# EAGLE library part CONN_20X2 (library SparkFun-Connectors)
Multi connection point. Often used as Generic Header-pin footprint for 0.1 inch spaced/style header connections On any of the 0.1 inch spaced packages, you can populate with these: Break Away Headers - Straight (PRT-00116) Break Away Male Headers - Right Angle (PRT-00553) Female Headers (PRT-00115) Break Away Headers - Machine Pin (PRT-00117) Break Away Female Headers - Swiss Machine Pin (PRT-00743)
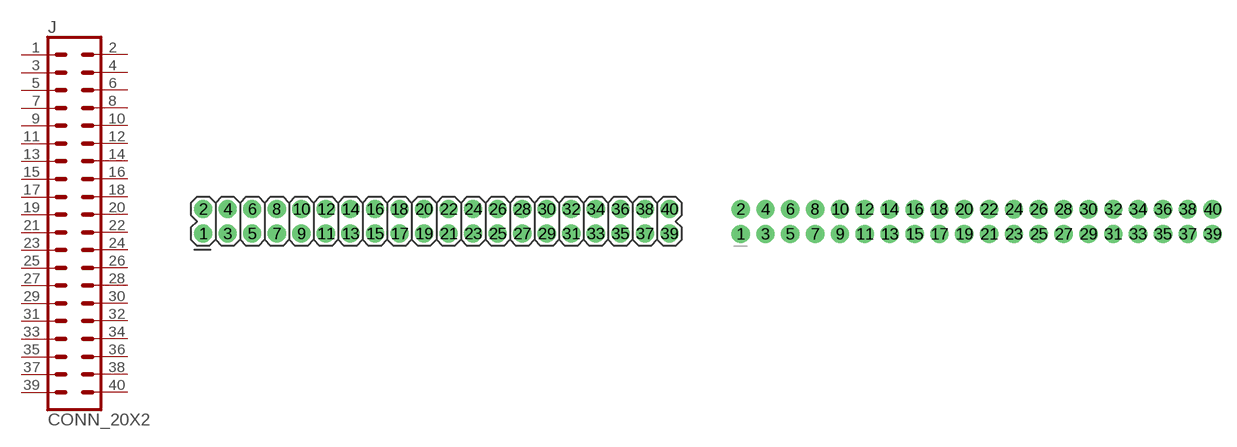
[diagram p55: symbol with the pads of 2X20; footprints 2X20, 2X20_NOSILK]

Designator prefix J

## CONN_20X2  [2X20]
1  1  pas
2  2  pas
3  3  pas
4  4  pas
5  5  pas
6  6  pas
7  7  pas
8  8  pas
9  9  pas
10  10  pas
11  11  pas
12  12  pas
13  13  pas
14  14  pas
15  15  pas
16  16  pas
17  17  pas
18  18  pas
19  19  pas
20  20  pas
21  21  pas
22  22  pas
23  23  pas
24  24  pas
25  25  pas
26  26  pas
27  27  pas
28  28  pas
29  29  pas
30  30  pas
31  31  pas
32  32  pas
33  33  pas
34  34  pas
35  35  pas
36  36  pas
37  37  pas
38  38  pas
39  39  pas
40  40  pas

## CONN_20X2NOSILK  [2X20_NOSILK]
Pads as for 2X20

## CONN_20X2SHROUDED (PROD_ID: CONN-12263; SF_ID: CONN-12263)  [2X20_SHROUDED]
Pads as for 2X20

## CONN_20X2SHROUDED_SMT (PROD_ID: CONN-13143)  [2X20_SHROUDED_SMT]
Pads as for 2X20

## Footprint 2X20 (pad centres in mm)
Plated Through Hole - 2x20 Specifications: Pin count:40 Pin pitch:0.1" Example device(s): CONN_20x2
drill 1.016 pad 1.88: 1 0,0; 2 0,2.54; 3 2.54,0; 4 2.54,2.54; 5 5.08,0; 6 5.08,2.54; 7 7.62,0; 8 7.62,2.54; 9 10.16,0; 10 10.16,2.54; 11 12.7,0; 12 12.7,2.54; 13 15.24,0; 14 15.24,2.54; 15 17.78,0; 16 17.78,2.54; 17 20.32,0; 18 20.32,2.54; 19 22.86,0; 20 22.86,2.54; 21 25.4,0; 22 25.4,2.54; 23 27.94,0; 24 27.94,2.54; 25 30.48,0; 26 30.48,2.54; 27 33.02,0; 28 33.02,2.54; 29 35.56,0; 30 35.56,2.54; 31 38.1,0; 32 38.1,2.54; 33 40.64,0; 34 40.64,2.54; 35 43.18,0; 36 43.18,2.54; 37 45.72,0; 38 45.72,2.54; 39 48.26,0; 40 48.26,2.54

## Footprint 2X20_NOSILK (pad centres in mm)
Plated Through Hole - 2x20 No Silk Outline Specifications: Pin count:40 Pin pitch:0.1" Example device(s): CONN_20x2
drill 1.016 pad 1.88: 1 0,0; 2 0,2.54; 3 2.54,0; 4 2.54,2.54; 5 5.08,0; 6 5.08,2.54; 7 7.62,0; 8 7.62,2.54; 9 10.16,0; 10 10.16,2.54; 11 12.7,0; 12 12.7,2.54; 13 15.24,0; 14 15.24,2.54; 15 17.78,0; 16 17.78,2.54; 17 20.32,0; 18 20.32,2.54; 19 22.86,0; 20 22.86,2.54; 21 25.4,0; 22 25.4,2.54; 23 27.94,0; 24 27.94,2.54; 25 30.48,0; 26 30.48,2.54; 27 33.02,0; 28 33.02,2.54; 29 35.56,0; 30 35.56,2.54; 31 38.1,0; 32 38.1,2.54; 33 40.64,0; 34 40.64,2.54; 35 43.18,0; 36 43.18,2.54; 37 45.72,0; 38 45.72,2.54; 39 48.26,0; 40 48.26,2.54

## Footprint 2X20_SHROUDED (pad centres in mm)
Plated Through Hole - 2x20 Shrouded Header Specifications: Pin count:40 Pin pitch:0.1" Datasheet referenced for footprint Example device(s): CONN_20x2
drill 1.016 pad 1.88: 1 -1.27,24.13; 2 1.27,24.13; 3 -1.27,21.59; 4 1.27,21.59; 5 -1.27,19.05; 6 1.27,19.05; 7 -1.27,16.51; 8 1.27,16.51; 9 -1.27,13.97; 10 1.27,13.97; 11 -1.27,11.43; 12 1.27,11.43; 13 -1.27,8.89; 14 1.27,8.89; 15 -1.27,6.35; 16 1.27,6.35; 17 -1.27,3.81; 18 1.27,3.81; 19 -1.27,1.27; 20 1.27,1.27; 21 -1.27,-1.27; 22 1.27,-1.27; 23 -1.27,-3.81; 24 1.27,-3.81; 25 -1.27,-6.35; 26 1.27,-6.35; 27 -1.27,-8.89; 28 1.27,-8.89; 29 -1.27,-11.43; 30 1.27,-11.43; 31 -1.27,-13.97; 32 1.27,-13.97; 33 -1.27,-16.51; 34 1.27,-16.51; 35 -1.27,-19.05; 36 1.27,-19.05; 37 -1.27,-21.59; 38 1.27,-21.59; 39 -1.27,-24.13; 40 1.27,-24.13

## Footprint 2X20_SHROUDED_SMT (pad centres in mm)
Surface Mount - 2x20 Shrouded Header Specifications: Pin count:40 Pin pitch:0.1" Datasheet referenced for footprint Example device(s): CONN_20x2
smd 4.14 x 0.991: 1 -3.569,24.13; 2 3.569,24.13; 3 -3.569,21.59; 4 3.569,21.59; 5 -3.569,19.05; 6 3.569,19.05; 7 -3.569,16.51; 8 3.569,16.51; 9 -3.569,13.97; 10 3.569,13.97; 11 -3.569,11.43; 12 3.569,11.43; 13 -3.569,8.89; 14 3.569,8.89; 15 -3.569,6.35; 16 3.569,6.35; 17 -3.569,3.81; 18 3.569,3.81; 19 -3.569,1.27; 20 3.569,1.27; 21 -3.569,-1.27; 22 3.569,-1.27; 23 -3.569,-3.81; 24 3.569,-3.81; 25 -3.569,-6.35; 26 3.569,-6.35; 27 -3.569,-8.89; 28 3.569,-8.89; 29 -3.569,-11.43; 30 3.569,-11.43; 31 -3.569,-13.97; 32 3.569,-13.97; 33 -3.569,-16.51; 34 3.569,-16.51; 35 -3.569,-19.05; 36 3.569,-19.05; 37 -3.569,-21.59; 38 3.569,-21.59; 39 -3.569,-24.13; 40 3.569,-24.13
